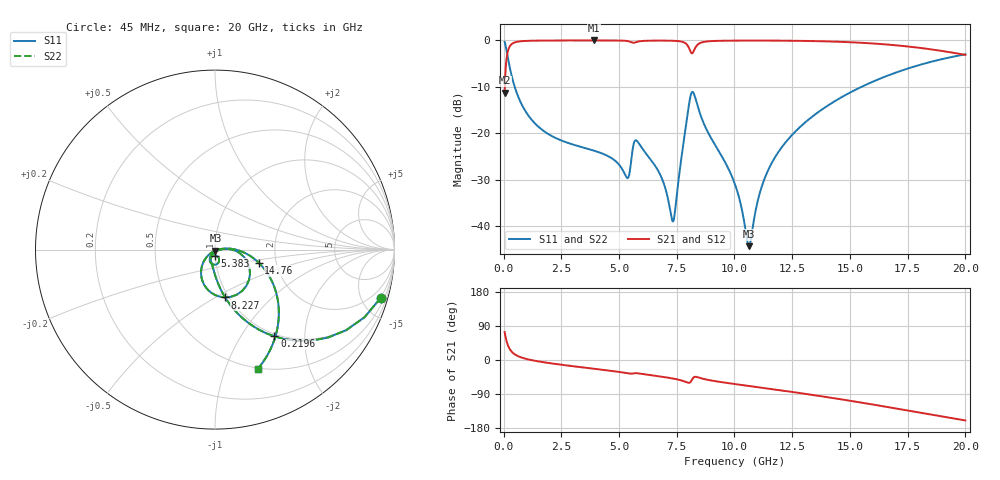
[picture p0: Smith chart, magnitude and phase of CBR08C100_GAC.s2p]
! S-parameter model data by Modelithics Inc.  support@modelithics.com 813-866-6335  Tampa FL USA
! S-Parameter data specifications:
! Substrate: 20-mil Rogers 4350B, substrate thickness, H=0.508mm, Dielectric constant, Er=3.75
! PCB Mounting Pad Footprint: Pad width, PadW=1.45mm , Pad length, PadL=1mm , Pad gap, PadG (edge-to-edge)=0.6mm , Reference planes=2.6mm apart
#  GHz  S  MA  R 50
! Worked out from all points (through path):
!   801 points, 45 MHz to 20 GHz, reference 50 ohm
!   highest |S21| = -0.04 dB at 3.911 GHz (marker M1); lowest = -11.3 dB at 45 MHz (marker M2)
!   group delay of S21, straight-line fit = 23 ps
!   lowest |S11| = -44.3 dB at 10.62 GHz (marker M3), VSWR 1.01, Z = 50.2 - j0.575 ohm
!   |S11| at or under -10 dB: 481.3 MHz to 15.5 GHz (15.02 GHz wide, 188 % of centre)
!   |S22| runs from -44.3 to -0.3 dB; largest |S21 - S12| = 0
!   S11 on the Smith chart (normalised r, x): 45 MHz: 0.96, -6.90; 219.6 MHz: 0.96, -1.42; 5.383 GHz: 1.00, -0.07; 8.227 GHz: 0.96, -0.55; 14.76 GHz: 1.62, -0.25; 20 GHz: 0.49, -1.30
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0.045  0.9619 -16.2  0.2734 73.8  0.2734 73.8  0.9619 -16.2
0.219606  0.5857 -55.6  0.8102 34.3  0.8102 34.3  0.5857 -55.6
0.344325  0.42 -67.5  0.907 22.4  0.907 22.4  0.42 -67.5
0.493988  0.309 -75.3  0.9504 14.6  0.9504 14.6  0.309 -75.3
1.2423  0.1375 -90.4  0.9895 -0.7  0.9895 -0.7  0.1375 -90.4
3.387462  0.07107 -108.1  0.9956 -19.3  0.9956 -19.3  0.07107 -108.1
3.911281  0.06515 -111.6  0.9957 -23.1  0.9957 -23.1  0.06515 -111.6
5.382962  0.03304 -89.0  0.9796 -35.1  0.9796 -35.1  0.03304 -89.0
5.732175  0.08433 -93.8  0.9534 -34.7  0.9534 -34.7  0.08433 -93.8
6.704981  0.03919 -123.4  0.992 -42.9  0.992 -42.9  0.03919 -123.4
7.353519  0.01143 -52.3  0.9878 -49.1  0.9878 -49.1  0.01143 -52.3
8.002056  0.1842 -18.7  0.8536 -60.1  0.8536 -60.1  0.1842 -18.7
8.22655  0.2719 -78.3  0.7584 -46.2  0.7584 -46.2  0.2719 -78.3
8.525875  0.1581 -119.3  0.9381 -47.7  0.9381 -47.7  0.1581 -119.3
10.0225  0.02826 -139.1  0.9916 -63.5  0.9916 -63.5  0.02826 -139.1
10.62115  0.006127 -69.2  0.9928 -68.5  0.9928 -68.5  0.006127 -69.2
11.09508  0.02277 2.7  0.9928 -72.4  0.9928 -72.4  0.02277 2.7
11.54407  0.04445 6.4  0.9921 -76.2  0.9921 -76.2  0.04445 6.4
13.36496  0.151 -4.3  0.9812 -92.0  0.9812 -92.0  0.151 -4.3
14.76181  0.2544 -16.7  0.959 -105.2  0.959 -105.2  0.2544 -16.7
16.68248  0.4215 -35.7  0.8975 -124.6  0.8975 -124.6  0.4215 -35.7
20  0.7061 -70.3  0.6967 -159.5  0.6967 -159.5  0.7061 -70.3
